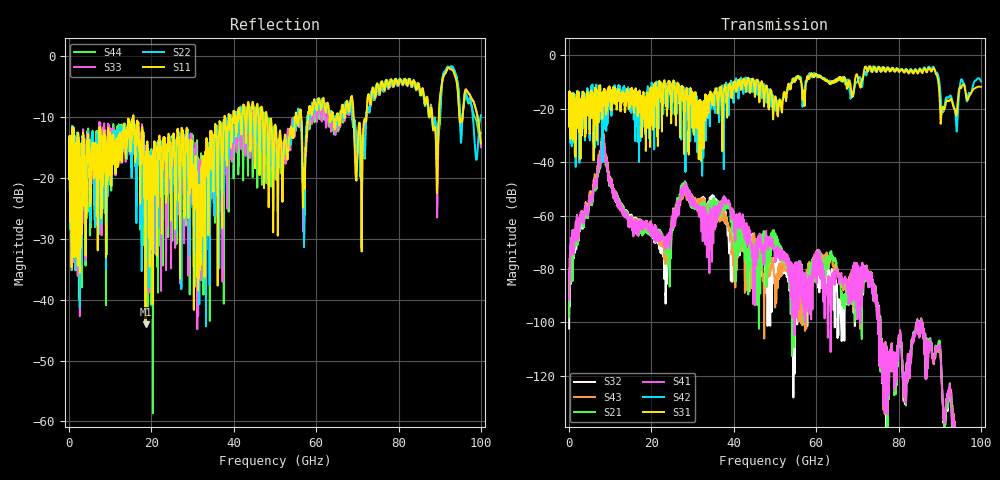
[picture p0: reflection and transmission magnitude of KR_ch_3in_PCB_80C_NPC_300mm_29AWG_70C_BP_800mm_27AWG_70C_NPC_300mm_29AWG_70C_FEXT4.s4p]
# GHz S RI R 45
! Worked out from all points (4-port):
!   4000 points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, 25 MHz to 100 GHz, reference 45 ohm
!   strongest paths, dB at 25 MHz, 25.02 GHz, 50.02 GHz, 75.03 GHz, 100 GHz:
!     S31: -20.0, -14.3, -16.0, -5.1, -11.8
!     S42: -20.0, -17.9, -18.0, -4.4, -9.7
!     S41: -90.7, -61.9, -76.3, -101.3, -180.0
!     S21: -97.9, -63.6, -68.8, -100.4, -179.5
!     S43: -97.0, -61.6, -92.8, -101.3, -177.7
!     S32: -102.3, -62.2, -77.6, -100.3, -178.3
!   lowest |S11| = -44.1 dB at 18.57 GHz (marker M1), VSWR 1.01, Z = 45.5 + j0.247 ohm
!   |S11| at or under -10 dB: start of sweep to 15.61 GHz; 15.64 GHz to 37.74 GHz (22.1 GHz wide, 82.8 % of centre); 48.05 GHz to 54.87 GHz (6.811 GHz wide, 13.2 % of centre)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
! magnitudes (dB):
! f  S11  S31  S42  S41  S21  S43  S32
! 25 MHz  -16.0  -20.0  -20.0  -90.7  -97.9  -97.0  -102.3
! 8.2 GHz  -18.1  -17.7  -28.5  -31.2  -33.0  -29.3  -30.8
! 18.57 GHz  -44.1  -20.9  -22.5  -62.8  -65.0  -62.9  -63.3
! 23.6 GHz  -24.1  -19.1  -12.8  -68.0  -70.0  -71.4  -78.2
! 27.95 GHz  -24.9  -37.0  -13.6  -50.7  -49.8  -51.7  -50.9
! 45.77 GHz  -7.9  -9.1  -14.7  -75.9  -84.8  -70.1  -78.8
! 100 GHz  -14.3  -11.8  -9.7  -180.0  -179.5  -177.7  -178.3
